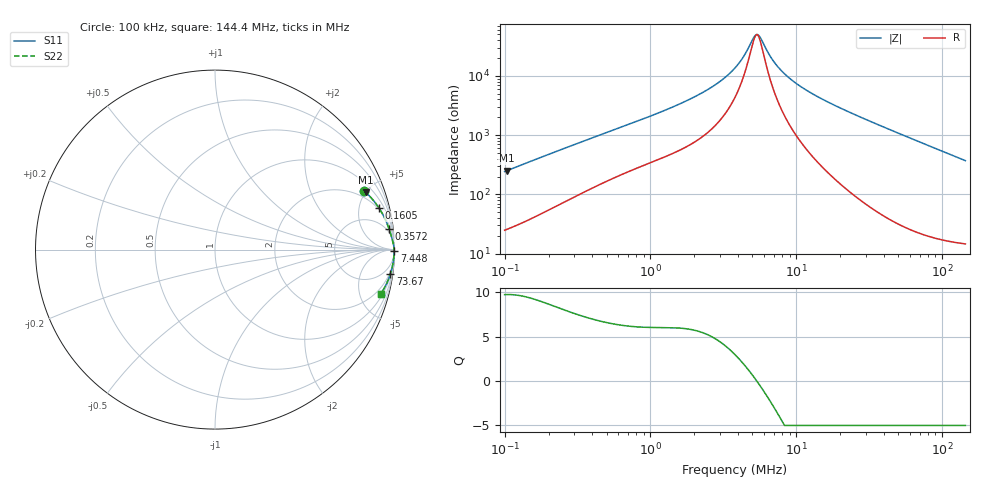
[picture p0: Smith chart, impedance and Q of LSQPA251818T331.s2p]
! LSQPA251818T331  S-PARAMETER MODEL  ( General Type )
! Model Generated by TAIYO YUDEN Corporation (http://www.ty-top.com)
! Version 3.0
! TAIYO YUDEN Control No. 160907NF25SB-FAC
! Copyright(c) 2007 TAIYO YUDEN CO.,LTD. All Rights Reserved.
! Product Description (link to TY-COMPAS)
! https://ds.yuden.co.jp/TYCOMPAS/or/detail?pn=LSQPA251818T331K&u=M
! Products Name : Inductors
! Characteristics :
!  Inductance : 330 uH , SRF(min) : 4.5 MHz , DC Resistance(max) : 15.99 Ohm
!  Rated Current : Saturation :100 mA , Temp Rise : 90 mA (40 degC)
!  Case Size : 2.5 x 1.8 / 0.098 x 0.071 [mm/inch] , Thickness : 1.8 / 0.071 [mm/inch]
!  (Conditions: Temperature = 25 degC , DC Bias Current/Voltage = 0A / 0V)
! External Node Assignments :
!  1  o---GGG---o  2
! GND o---------o GND
! Frequency Range : 0.1MHz  -  144.390904MHz  [ 402 STEP ]
# MHz S RI R 50
! Freq[MHz].  S11 Real  S11 Imag  S21 Real  S21 Imag  S12 Real  S12 Imag  S22 Real  S22 Imag
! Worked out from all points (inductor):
!   401 points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, 100 kHz to 144.4 MHz, reference 50 ohm
!   read as one part in series: L = 381 uH near 103.7 kHz
!   highest Q = 9.73 at 103.7 kHz (marker M1), where L = 383 uH
!   self-resonance near 5.272 MHz
!   S11 on the Smith chart (normalised r, x): 100 kHz: 1.50, +4.82; 160.5 kHz: 1.83, +7.61; 357.2 kHz: 3, +16; 7.448 MHz: open; 73.67 MHz: 1, -15; 144.4 MHz: 1.29, -7.40
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0.1  0.8305 0.3273  0.1695 -0.3273  0.1695 -0.3273  0.8305 0.3273
0.103705  0.8392 0.3196  0.1608 -0.3196  0.1608 -0.3196  0.8392 0.3196
0.160461  0.9143 0.2309  0.0857 -0.2309  0.0857 -0.2309  0.9143 0.2309
0.338238  0.9674 0.1221  0.0326 -0.1221  0.0326 -0.1221  0.9674 0.1221
0.357207  0.9694 0.1164  0.0306 -0.1164  0.0306 -0.1164  0.9694 0.1164
1.144052  0.9915 0.0407  0.00848 -0.0407  0.00848 -0.0407  0.9915 0.0407
1.770183  0.995 0.0257  0.00505 -0.0257  0.00505 -0.0257  0.995 0.0257
2.455826  0.9965 0.0168  0.0035 -0.0168  0.0035 -0.0168  0.9965 0.0168
3.167973  0.9973 0.0108  0.00275 -0.0108  0.00275 -0.0108  0.9973 0.0108
3.869624  0.9976 0.00656  0.00236 -0.00656  0.00236 -0.00656  0.9976 0.00656
4.395019  0.9978 0.00396  0.00218 -0.00396  0.00218 -0.00396  0.9978 0.00396
5.083368  0.998 0.00106  0.00204 -0.00106  0.00204 -0.00106  0.998 0.00106
5.368439  0.998 -2.89e-05  0.002 2.89e-05  0.002 2.89e-05  0.998 -2.89e-05
5.669498  0.998 -0.00112  0.00196 0.00112  0.00196 0.00112  0.998 -0.00112
6.557456  0.9981 -0.00404  0.0019 0.00404  0.0019 0.00404  0.9981 -0.00404
7.447789  0.9981 -0.00668  0.00188 0.00668  0.00188 0.00668  0.9981 -0.00668
9.434359  0.9981 -0.0119  0.00192 0.0119  0.00192 0.0119  0.9981 -0.0119
12.85266  0.9979 -0.0198  0.00214 0.0198  0.00214 0.0198  0.9979 -0.0198
20.62353  0.9969 -0.0358  0.00311 0.0358  0.00311 0.0358  0.9969 -0.0358
43.47261  0.9912 -0.0793  0.00878 0.0793  0.00878 0.0793  0.9912 -0.0793
73.6686  0.9778 -0.1337  0.0222 0.1337  0.0222 0.1337  0.9778 -0.1337
144.3909  0.9236 -0.2467  0.0764 0.2467  0.0764 0.2467  0.9236 -0.2467
